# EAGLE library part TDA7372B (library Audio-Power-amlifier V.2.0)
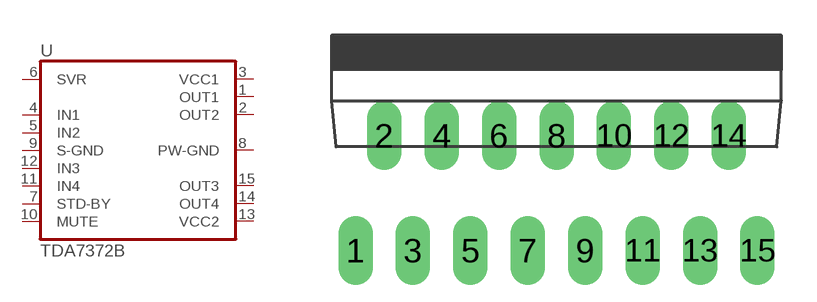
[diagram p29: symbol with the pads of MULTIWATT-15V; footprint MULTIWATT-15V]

Designator prefix -

## TDA7372B  [MULTIWATT-15V]
1  OUT1  out
2  OUT2  out
3  VCC1  pwr
4  IN1  in
5  IN2  in
6  SVR  pas
7  STD-BY  in
8  PW-GND  pwr
9  S-GND  in
10  MUTE  in
11  IN4  in
12  IN3  in
13  VCC2  pwr
14  OUT4  out
15  OUT3  out

## Footprint MULTIWATT-15V (pad centres in mm)
Multiwatt 15 vertical
drill 1.016 long: 1 -8.89,-5.08; 2 -7.62,0; 3 -6.35,-5.08; 4 -5.08,0; 5 -3.81,-5.08; 6 -2.54,0; 7 -1.27,-5.08; 8 0,0; 9 1.27,-5.08; 10 2.54,0; 11 3.81,-5.08; 12 5.08,0; 13 6.35,-5.08; 14 7.62,0; 15 8.89,-5.08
